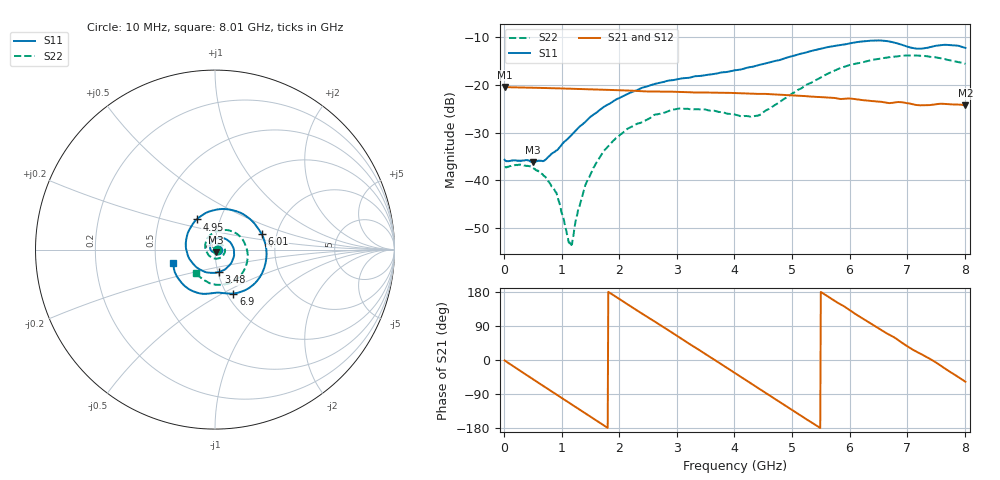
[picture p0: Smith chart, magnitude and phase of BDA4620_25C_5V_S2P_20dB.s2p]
!Agilent Technologies,E5071B,MY42404982,A.09.10
!Date: Wed May 06 09:02:36 2026
!Data & Calibration Information:
!Freq	S11:SOLT2(ON)	S21:SOLT2(ON)	S12:SOLT2(ON)	S22:SOLT2(ON)
# Hz S RI R 50
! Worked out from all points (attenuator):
!   801 points, 10 MHz to 8.01 GHz, reference 50 ohm
!   highest |S21| = -20.41 dB at 10 MHz (marker M1); lowest = -24.3 dB at 8.01 GHz (marker M2)
!   lowest |S11| = -36.1 dB at 500 MHz (marker M3), VSWR 1.03, Z = 50.3 - j1.52 ohm
!   |S11| at or under -10 dB: start of sweep to end of sweep
!   |S22| runs from -53.8 to -13.8 dB; largest |S21 - S12| = 0.0004
!   S11 on the Smith chart (normalised r, x): 10 MHz: 1.03, -0.00; 3.48 GHz: 1.01, -0.26; 4.95 GHz: 0.77, +0.27; 6.01 GHz: 1.66, +0.31; 6.9 GHz: 1.07, -0.57; 8.01 GHz: 0.62, -0.10
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1e7  0.0164 -0.00118  0.0954 -0.00202  0.0955 -0.00203  0.0137 -0.000453
5e8  0.0037 -0.0151  0.0597 -0.0722  0.0598 -0.0724  0.0124 -0.00553
7e8  -0.00715 -0.0145  0.0312 -0.0877  0.0312 -0.0879  0.00865 -0.00701
8.9e8  -0.0181 -0.00884  0.00112 -0.0925  0.001 -0.0926  0.00384 -0.00661
1.15e9  -0.0274 0.00933  -0.0389 -0.0829  -0.0391 -0.0831  -0.00172 -0.00111
1.19e9  -0.028 0.013  -0.0445 -0.0798  -0.0446 -0.08  -0.00239 0.000133
1.35e9  -0.0269 0.0273  -0.0642 -0.0643  -0.0642 -0.0643  -0.00399 0.00521
1.54e9  -0.0182 0.0448  -0.0807 -0.0399  -0.0808 -0.04  -0.00358 0.0125
1.77e9  0.00253 0.0607  -0.089 -0.00584  -0.0891 -0.00585  0.000782 0.0215
2.15e9  0.0521 0.0621  -0.073 0.0485  -0.0731 0.0486  0.0179 0.0301
2.68e9  0.105 0.00024  -0.00771 0.0852  -0.00759 0.0853  0.0457 0.019
3.48e9  0.0209 -0.1251  0.0799 0.025  0.08 0.025  0.0399 -0.0387
4.01e9  -0.1047 -0.0972  0.0679 -0.0467  0.068 -0.0469  -0.0122 -0.0476
4.42e9  -0.1616 0.00791  0.0214 -0.078  0.0213 -0.0781  -0.0467 -0.0125
4.95e9  -0.1024 0.1681  -0.047 -0.0626  -0.0471 -0.0627  -0.0378 0.0676
5.35e9  0.0358 0.2261  -0.0733 -0.0184  -0.0735 -0.0185  0.0234 0.1046
6.01e9  0.2597 0.0872  -0.047 0.055  -0.0471 0.0551  0.1512 0.0603
6.35e9  0.2825 -0.0715  -0.00912 0.0677  -0.00911 0.0678  0.1803 -0.0118
6.68e9  0.195 -0.2107  0.0248 0.0598  0.025 0.06  0.172 -0.0925
6.9e9  0.1025 -0.2449  0.0456 0.0479  0.0457 0.0481  0.1454 -0.1415
7.56e9  -0.1088 -0.2367  0.062 -0.0139  0.0622 -0.014  -0.0156 -0.1912
8.01e9  -0.2329 -0.0754  0.0331 -0.0515  0.0333 -0.0516  -0.1064 -0.1279
